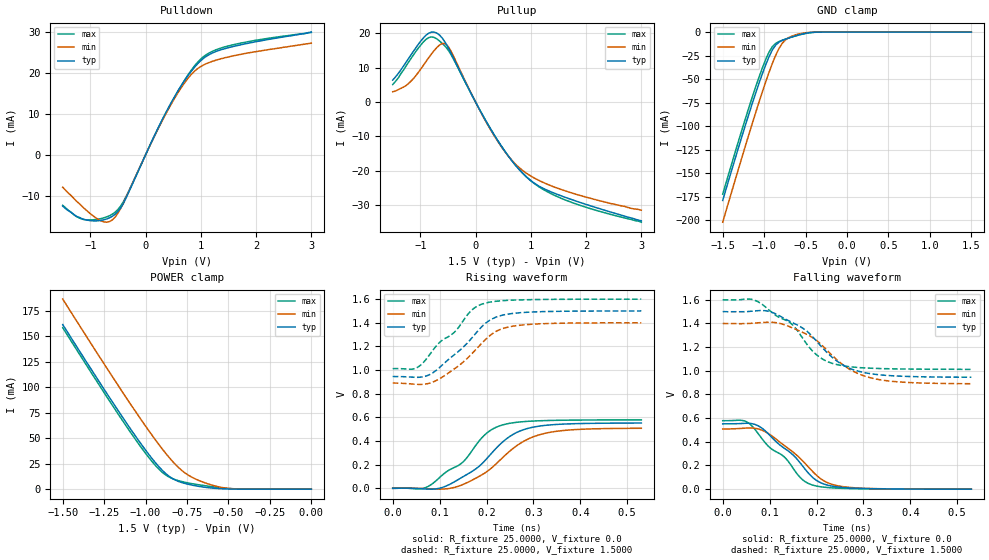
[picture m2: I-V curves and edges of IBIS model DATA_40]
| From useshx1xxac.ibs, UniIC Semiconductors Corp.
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|   Model DATA_40
[Model]  DATA_40
Model_type   I/O
Polarity   Non-Inverting
Enable   Active-High
Vinl =   0.600000V
Vinh =   0.900000V
Vmeas =   0.750000V
Rref =   25.000000
Vref =   0.7500000V
C_comp   1.3900pF   1.3640pF   1.5600pF
[Temperature Range]   25.0000   95.0000   0.0
[Voltage Range]   1.5000V   1.4000V   1.6000V
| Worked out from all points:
|   slope of the pulldown table from 0 to 0.225 V, typ, clamps not added: 34.7 ohm
|   slope of the pullup table from 0 to 0.225 V, typ, clamps not added: 34.4 ohm
|   GND clamp passes 1 mA (typ) near -0.48 V on its own axis
|   POWER clamp passes 1 mA (typ) near -0.59 V on its own axis
|   rising waveform, R_fixture 25.0000, V_fixture 0.0: 20-80 % time 95.5ps typ, 98.7ps min, 92.5ps max; typ from 0 V to 0.552 V
|   rising waveform, R_fixture 25.0000, V_fixture 1.5000: 20-80 % time 86.4ps typ, 84.2ps min, 84.1ps max; typ from 0.946 V to 1.5 V
|   falling waveform, R_fixture 25.0000, V_fixture 0.0: 20-80 % time 85.1ps typ, 85.4ps min, 84.6ps max; typ from 0.552 V to 0 V
|   falling waveform, R_fixture 25.0000, V_fixture 1.5000: 20-80 % time 95.2ps typ, 95.9ps min, 93.5ps max; typ from 1.5 V to 0.946 V
[Pulldown]
|Voltage   I(typ)   I(min)   I(max)
-1.5V     -12.5mA    -7.9mA     -12.3mA
-1.1V     -15.78mA   -13.18mA   -15.82mA
-800mV    -15.97mA   -16.14mA   -15.52mA
-650mV    -15.34mA   -16.26mA   -14.83mA
-550mV    -14.48mA   -15.16mA   -13.97mA
-400mV    -11.78mA   -11.73mA   -11.39mA
400mV     11.12mA    10.81mA    10.96mA
650mV     16.95mA    16.45mA    16.95mA
900mV     21.56mA    20.54mA    21.89mA
1.15V     24.41mA    22.48mA    24.81mA
1.45V     25.92mA    23.69mA    26.35mA
3V        29.9mA     27.2mA     29.8mA
[Pullup]
|Voltage   I(typ)   I(min)   I(max)
-1.5V     6.4mA      3mA        5.1mA
-1.2V     12.96mA    5.6mA      11.91mA
-850mV    20mA       12.86mA    18.73mA
-700mV    20.03mA    15.87mA    18.36mA
-550mV    17.36mA    16.99mA    16.21mA
-450mV    14.37mA    14.95mA    13.96mA
300mV     -8.588mA   -8.811mA   -8.555mA
550mV     -14.74mA   -14.81mA   -14.71mA
800mV     -19.76mA   -19.19mA   -19.78mA
1.1V      -23.96mA   -22.39mA   -24.11mA
1.55V     -27.24mA   -25.4mA    -27.96mA
3V        -34.5mA    -31.4mA    -34.9mA
[GND_clamp]
|Voltage   I(typ)   I(min)   I(max)
-1.5V     -178.7mA   -201.8mA   -172.1mA
-1.18V    -85.9mA    -107.5mA   -79.02mA
-1.06V    -53.85mA   -73.82mA   -47.38mA
-980mV    -34.46mA   -52.52mA   -28.79mA
-940mV    -25.94mA   -42.47mA   -21.09mA
-900mV    -18.8mA    -33.04mA   -15.34mA
-860mV    -13.68mA   -24.5mA    -11.91mA
-780mV    -8.804mA   -11.75mA   -8.617mA
-740mV    -7.413mA   -8.071mA   -7.384mA
-620mV    -3.934mA   -2.917mA   -4.046mA
-420mV    -302.4uA   -187.9uA   -428.5uA
1.5V      1.623nA    17.64nA    1.98nA
[POWER_clamp]
|Voltage   I(typ)   I(min)   I(max)
-1.5V     161.3mA    186.3mA    158.3mA
-1.22V    90.37mA    115.2mA    87.1mA
-1.04V    47.2mA     71.18mA    43.94mA
-980mV    33.96mA    57.17mA    30.91mA
-920mV    22.07mA    43.79mA    19.67mA
-880mV    15.49mA    35.42mA    14.07mA
-840mV    10.61mA    27.72mA    10.46mA
-780mV    6.409mA    18.15mA    7.405mA
-720mV    3.991mA    11.66mA    5.381mA
-560mV    586.1uA    2.318mA    1.645mA
-440mV    47uA       184.9uA    218uA
0V        1.623nA    5.301nA    2.263nA
[Ramp]
| variable   typ   min   max
dV/dt_r  0.3315/96.9880p   0.3052/0.1003n   0.3474/93.1896p
dV/dt_f  0.3332/96.7909p   0.3063/97.5091p   0.3528/94.6531p
R_load = 25.0000
[Rising Waveform]
R_fixture= 25.0000
V_fixture= 0.0
V_fixture_min= 0.0
V_fixture_max= 0.0
|time   V(typ)   V(min)   V(max)
0s        0V         0V         0V
65ps      -4.097mV   -2.199mV   -641.6uV
115ps     21.52mV    -3.854mV   141.1mV
150ps     98.23mV    32.69mV    223.2mV
180ps     172.9mV    91.67mV    379.1mV
205ps     270.9mV    153.7mV    480.8mV
235ps     394mV      262.1mV    536.7mV
280ps     497.2mV    399.2mV    564.1mV
330ps     534.1mV    469.4mV    573.2mV
530ps     551.8mV    507.6mV    578.7mV
[Rising Waveform]
R_fixture= 25.0000
V_fixture= 1.5000
V_fixture_min= 1.4000
V_fixture_max= 1.6000
|time   V(typ)   V(min)   V(max)
0s        945.6mV    890.9mV    1.012V
50ps      938.4mV    879.5mV    1.017V
80ps      963.9mV    890.6mV    1.137V
100ps     1.022V     926.7mV    1.234V
140ps     1.157V     1.034V     1.358V
170ps     1.277V     1.143V     1.512V
195ps     1.386V     1.247V     1.563V
225ps     1.454V     1.336V     1.583V
265ps     1.482V     1.376V     1.592V
530ps     1.5V       1.4V       1.6V
[Falling Waveform]
R_fixture= 25.0000
V_fixture= 0.0
V_fixture_min= 0.0
V_fixture_max= 0.0
|time   V(typ)   V(min)   V(max)
0s        551.8mV    507.6mV    578.7mV
50ps      556.7mV    516.2mV    570.9mV
80ps      525.2mV    503.7mV    446.2mV
100ps     456.3mV    463.1mV    352.6mV
135ps     335.7mV    357.9mV    257.8mV
170ps     197.3mV    240.8mV    80.49mV
195ps     88.23mV    136mV      30.96mV
225ps     32.55mV    52.26mV    13.28mV
265ps     11.65mV    17.14mV    5.682mV
530ps     0V         0V         0V
[Falling Waveform]
R_fixture= 25.0000
V_fixture= 1.5000
V_fixture_min= 1.4000
V_fixture_max= 1.6000
|time   V(typ)   V(min)   V(max)
0s        1.5V       1.4V       1.6V
65ps      1.504V     1.402V     1.6V
110ps     1.486V     1.408V     1.477V
150ps     1.404V     1.36V      1.384V
180ps     1.333V     1.306V     1.221V
205ps     1.228V     1.24V      1.12V
235ps     1.108V     1.124V     1.061V
275ps     1.014V     1.003V     1.033V
325ps     970.3mV    931.9mV    1.02V
530ps     945.6mV    890.9mV    1.012V
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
